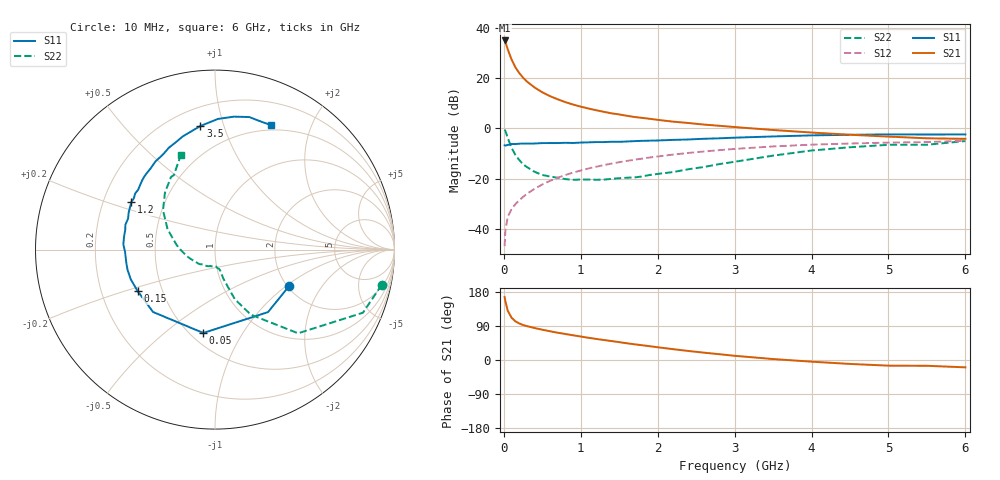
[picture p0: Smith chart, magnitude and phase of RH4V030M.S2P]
! SIEMENS Small Signal Semiconductors
! BFR106
! Si NPN RF Bipolar Junction Transistor in SOT23
! VCE = 4 V  IC = 30 mA
! Common Emitter S-Parameters:  August  1996
# GHz  S  MA  R  50
!  f  S11  S21  S12  S22
! GHz  MAG  ANG  MAG  ANG  MAG  ANG  MAG  ANG
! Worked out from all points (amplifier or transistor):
!   36 points, 10 MHz to 6 GHz, reference 50 ohm
!   highest |S21| = 35.1 dB at 10 MHz (marker M1)
!   |S21| within 3 dB of that: start of sweep to 45.11 MHz
!   unconditionally stable (mu >= 1): 307.8 MHz to 2.235 GHz
!   at 250 MHz: K = 0.95, MSG = 23.8 dB, |S12| = -27.3 dB
!   at 1.4 GHz: K = 1.06, MAG = 8.5 dB, |S12| = -14.0 dB
!   at 6 GHz: K = 0.99, MSG = 0.4 dB, |S12| = -4.9 dB
!   S11 on the Smith chart (normalised r, x): 10 MHz: 2.06, -1.05; 50 MHz: 0.58, -0.69; 150 MHz: 0.36, -0.22; 1.2 GHz: 0.32, +0.24; 3.5 GHz: 0.32, +0.84; 6 GHz: 0.44, +1.46
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0.01  0.4609 -25.8  56.91 166.2  0.0045 81.7  0.9494 -11.9
0.02  0.4567 -49.7  52.71 154.9  0.009 72.9  0.8962 -23.1
0.05  0.469 -98.0  38.23 130.4  0.0173 60.0  0.6572 -45.2
0.1  0.4899 -134.8  23.74 111.6  0.0247 56.8  0.4134 -61.2
0.15  0.4891 -151.9  16.61 102.0  0.031 58.3  0.2976 -68.2
0.2  0.4977 -160.6  12.78 96.5  0.037 61.7  0.2356 -70.2
0.25  0.5001 -166.9  10.3 92.3  0.0432 63.6  0.1926 -72.3
0.3  0.4995 -171.4  8.644 89.4  0.0499 65.5  0.1702 -73.8
0.4  0.5014 -178.6  6.558 84.4  0.0627 67.7  0.1368 -75.3
0.5  0.5115 176.7  5.268 79.9  0.0765 68.7  0.1183 -76.2
0.6  0.5119 171.4  4.417 75.8  0.0902 68.8  0.1101 -78.2
0.7  0.5122 167.4  3.82 72.0  0.1039 68.7  0.1041 -81.9
0.9  0.514 160.4  3.002 65.2  0.1319 66.9  0.0946 -87.2
1.1  0.5289 153.7  2.502 58.7  0.1593 65.1  0.0959 -97.1
1.2  0.5356 150.5  2.311 55.6  0.1725 64.0  0.0949 -101.6
1.6  0.5501 139.5  1.789 44.1  0.2255 58.9  0.1042 -121.8
2.2  0.5927 124.0  1.369 28.6  0.3016 50.4  0.1351 -152.7
2.8  0.6365 110.1  1.132 15.3  0.3696 41.2  0.1948 179.4
3.5  0.6935 96.7  0.933 2.5  0.4385 30.6  0.2876 156.8
4.5  0.7482 81.9  0.75 -10.4  0.5014 15.7  0.4224 131.3
5.5  0.7578 69.9  0.637 -15.3  0.5359 5.8  0.4741 118.9
6  0.7608 65.7  0.622 -19.4  0.5684 -1.5  0.5612 109.8
